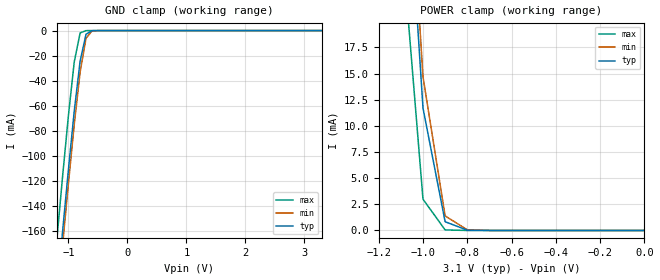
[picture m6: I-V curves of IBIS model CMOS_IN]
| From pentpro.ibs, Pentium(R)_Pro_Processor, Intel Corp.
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[Model]   CMOS_IN
Model_type  Input
Polarity   Inverting
Enable   Active-Low
Vinl = 0.8
Vinh = 2.0
|Variable   typ   min   max
C_comp   2.6p   2.3p   2.8p
|Variable   typ   min   max
[Voltage range] 3.1   2.845  3.255
|Variable   typ   min   max
[Temperature Range] 80   0   100
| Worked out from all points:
|   GND clamp passes 1 mA (typ) near -0.63 V on its own axis
|   POWER clamp passes 1 mA (typ) near -0.90 V on its own axis
[GND_clamp]
|Volts   typ   min   max
-3.3V     -1.36A     -1.38A     -1.3A
-1.2V     -214mA     -225mA     -170mA
-1.1V     -162mA     -173mA     -118mA
-1V       -112mA     -123mA     -68.7mA
-900mV    -64.5mA    -75.2mA    -25.1mA
-800mV    -24.3mA    -33.1mA    -1.87mA
-700mV    -2.93mA    -6.13mA    -28.1uA
-600mV    -120uA     -353uA     0A
3.3V      0A         0A         0A
[POWER_clamp]
|Volts   typ   min   max
-3.3V     1.19A      1.21A      1.19A
-1.1V     44.5mA     48.7mA     28.8mA
-1V       11.7mA     14.7mA     2.99mA
-900mV    835uA      1.39mA     53.6uA
-800mV    32.8uA     66.7uA     0A
0V        0A         0A         0A
